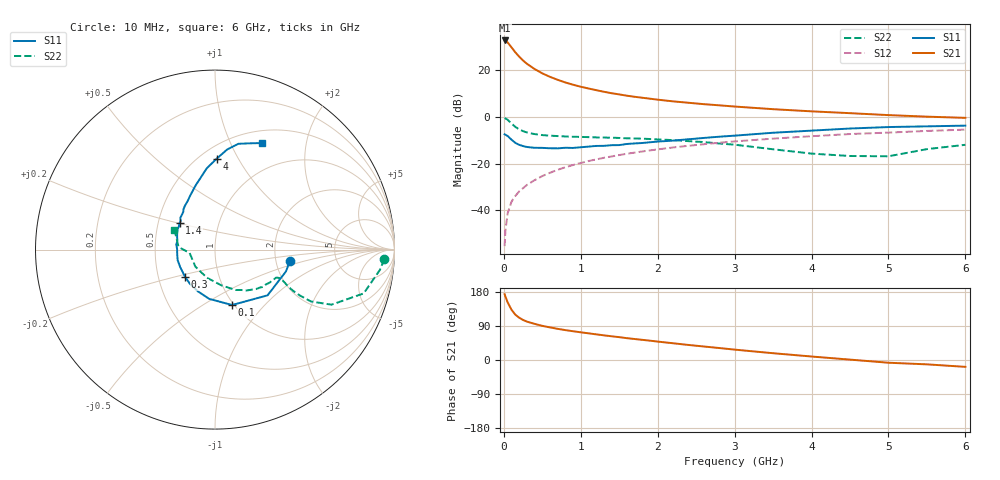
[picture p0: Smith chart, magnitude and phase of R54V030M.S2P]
! SIEMENS Small Signal Semiconductors
! BFR183
! Si NPN RF Bipolar Junction Transistor in SOT23
! VCE = 4 V  IC = 30 mA
! Common Emitter S-Parameters:  May  1996
# GHz  S  MA  R  50
!  f  S11  S21  S12  S22
! GHz  MAG  ANG  MAG  ANG  MAG  ANG  MAG  ANG
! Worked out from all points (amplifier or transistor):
!   36 points, 10 MHz to 6 GHz, reference 50 ohm
!   highest |S21| = 32.7 dB at 10 MHz (marker M1)
!   |S21| within 3 dB of that: start of sweep to 100.8 MHz
!   unconditionally stable (mu >= 1): 467.6 MHz to 2.353 GHz
!   at 250 MHz: K = 0.89, MSG = 27.3 dB, |S12| = -30.5 dB
!   at 1.4 GHz: K = 1.05, MAG = 12.2 dB, |S12| = -17.0 dB
!   at 6 GHz: K = 0.90, MSG = 2.5 dB, |S12| = -5.5 dB
!   S11 on the Smith chart (normalised r, x): 10 MHz: 2.39, -0.38; 100 MHz: 0.98, -0.68; 300 MHz: 0.69, -0.22; 1.4 GHz: 0.64, +0.20; 4 GHz: 0.60, +0.82; 6 GHz: 0.64, +1.32
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0.01  0.4222 -8.8  43.14 173.7  0.0017 85.5  0.9449 -3.2
0.02  0.4134 -17.2  42.75 167.7  0.0036 80.5  0.9259 -7.0
0.05  0.3882 -41.0  39.06 151.9  0.0087 76.8  0.8638 -16.4
0.1  0.3232 -72.8  30.66 132.5  0.0153 72.3  0.718 -25.3
0.15  0.2765 -96.7  23.96 119.5  0.0203 69.7  0.6079 -28.4
0.2  0.2512 -112.4  19.38 111.5  0.0253 71.5  0.5381 -28.4
0.25  0.2363 -126.4  16.04 105.7  0.0297 71.3  0.4922 -27.8
0.3  0.2259 -137.4  13.66 101.3  0.0348 72.3  0.4627 -27.0
0.4  0.2171 -153.1  10.55 95.3  0.0441 73.8  0.4267 -25.2
0.5  0.2163 -164.3  8.515 90.1  0.0539 74.3  0.4063 -24.1
0.6  0.2122 -172.8  7.177 86.0  0.0634 74.1  0.3946 -23.8
0.8  0.2175 172.7  5.439 78.9  0.0833 72.9  0.3797 -24.3
0.9  0.2155 166.7  4.861 75.9  0.093 72.3  0.3743 -24.7
1.1  0.23 156.5  4.04 70.4  0.1129 71.0  0.3671 -27.0
1.4  0.247 143.1  3.203 62.6  0.1417 68.0  0.3573 -30.5
1.7  0.269 132.7  2.685 55.4  0.1713 64.9  0.3428 -34.8
2.2  0.3094 119.7  2.143 44.2  0.2206 59.1  0.3173 -43.9
3.5  0.456 95.7  1.457 17.9  0.3411 42.4  0.2018 -80.1
4  0.5061 89.0  1.31 9.2  0.3843 36.4  0.163 -106.1
4.5  0.5616 83.1  1.197 1.0  0.4277 29.6  0.1449 -138.8
5.5  0.6249 71.4  1.008 -11.5  0.4983 17.8  0.2033 175.9
6  0.6477 66.4  0.95 -18.1  0.5319 10.3  0.2517 154.0
